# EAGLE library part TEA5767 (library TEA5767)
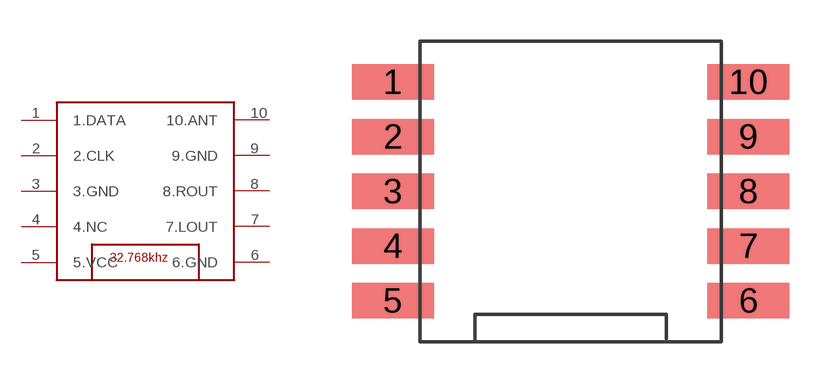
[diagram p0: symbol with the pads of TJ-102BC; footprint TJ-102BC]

Designator prefix -

## TEA5767  [TJ-102BC]
1  1.DATA
2  2.CLK
3  3.GND
4  4.NC
5  5.VCC
6  6.GND
7  7.LOUT
8  8.ROUT
9  9.GND
10  10.ANT

## Footprint TJ-102BC (pad centres in mm)
smd 3 x 1.3: 1 -2,0.5; 2 -2,-1.5; 3 -2,-3.5; 4 -2,-5.5; 5 -2,-7.5; 6 11,-7.5; 7 11,-5.5; 8 11,-3.5; 9 11,-1.5; 10 11,0.5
